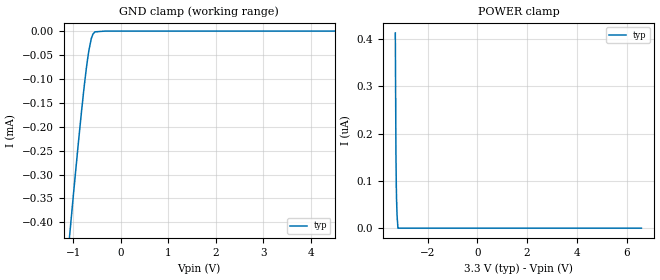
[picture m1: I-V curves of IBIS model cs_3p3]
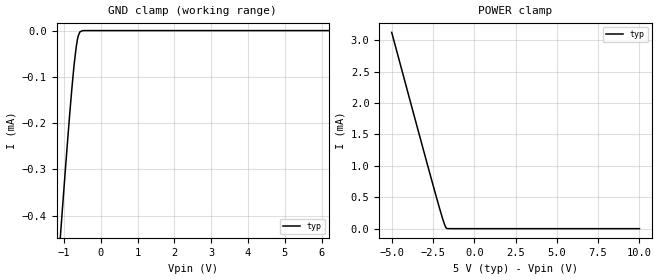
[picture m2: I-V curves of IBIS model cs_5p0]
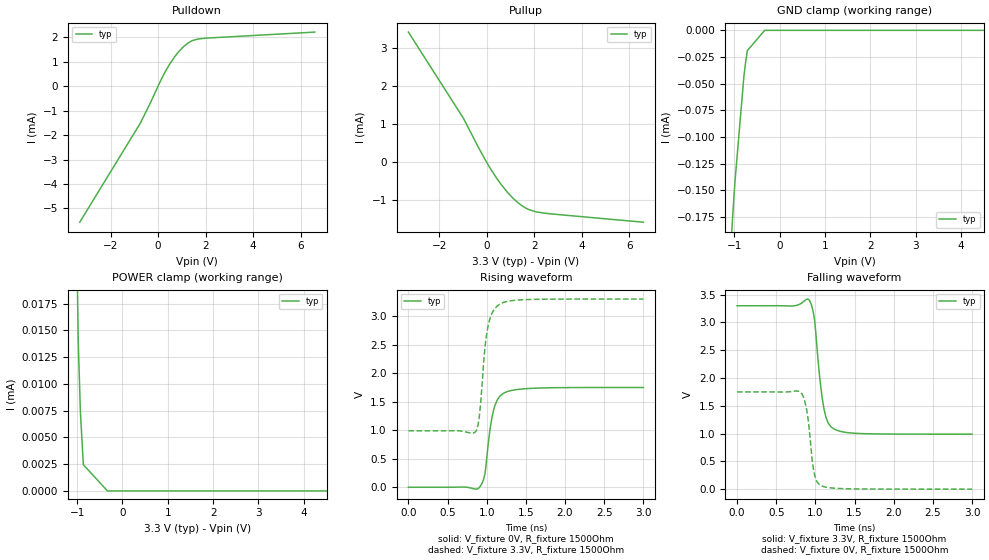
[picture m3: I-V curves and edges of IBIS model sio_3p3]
|Texas Instruments Incorporated
|LM70 SPI/MICROWIRE 10-Bit plus Sign Digital Temperature Sensor
|Marketing part#   Digital Voltage Range   Package-type   #pins
|LM70CIMM-3   2.65-5.5   VSSOP   8
|LM70CIMM-3/NOPB   2.65-5.5   VSSOP   8
|LM70CIMM-5   2.65-5.5   VSSOP   8
|LM70CIMM-5/NOPB   2.65-5.5   VSSOP   8
|LM70CIMMX-3   2.65-5.5   VSSOP   8
|LM70CIMMX-3/NOPB   2.65-5.5   VSSOP   8
|LM70CIMMX-5/NOPB   2.65-5.5   VSSOP   8
|LM70CILD-3/NOPB   2.65-5.5   WSON   8
|LM70CILD-5/NOPB   2.65-5.5   WSON   8
|LM70CILDX-3/NOPB   2.65-5.5   WSON   8
[IBIS Ver]   4.1
[File name]   lm70.ibs
[File Rev]   1.0
[Date]   10/25/2016
[Source]
| Texas Instruments Incorporated.
| Analog-eLab Design Center, HPA
| 12500 TI Blvd
| Dallas, TX -75243
[Notes]   Revision History:
| Rev 1.0: 10/25/2016
| - Initial version of the model
| - Model generated from simulations in SPECTRE
| - Model matched to SPICE simulation
| - C_comp although listed in numerical order of value are
|   obtained from varying PVT conditions. For PVT conditions for
|   each specific value refer the buffer description under
|   respective [Model]. IBIS model user is responsible for using
|   appropriate C_comp to simulate for Signal Integrity.
| - Only Typical corners are modeled.
[Disclaimer]
| This model is designed as an aid for customers of Texas Instruments.
| TI and its licensors and suppliers make no warranties, either expressed
| or implied, with respect to this  model, including the warranties of
| merchantability or fitness for a particular purpose. The model is
| provided solely on an "as is" basis. The entire risk as to its quality
| and performance is with the customer.
[Copyright]
(C) Copyright 2016 Texas Instruments Incorporated.All rights reserved.
|   LM70DGK
[Component]   LM70DGK
[Manufacturer]   TI
[Package]   |8 VSSOP - DGK Package
|   typ   min   max
R_pkg   0.5   na   na
L_pkg   1n   na   na
C_pkg   .5p   na   na
[Pin]  signal_name   model_name   R_pin   L_pin   C_pin
1   SI/O   sio   na   na   na
2   SC   cs   na   na   na
3   NC   nc   na   na   na
4   GND   gnd   na   na   na
5   V+   power   na   na   na
6   NC   nc   na   na   na
7   _CS   cs   na   na   na
8   NC   nc   na   na   na
|   LM70NGK
[Component]   LM70NGK
[Manufacturer]   TI
[Package]   |8 WSON - NGK Package
|   typ   min   max
R_pkg   0.5   na   na
L_pkg   1n   na   na
C_pkg   .5p   na   na
[Pin]  signal_name   model_name   R_pin   L_pin   C_pin
1   SI/O   sio   na   na   na
2   NC   nc   na   na   na
3   SC   cs   na   na   na
4   NC   nc   na   na   na
5   V+   power   na   na   na
6   NC   nc   na   na   na
7   GND   gnd   na   na   na
8   _CS   cs   na   na   na
|   Model Selectors
[Model Selector] cs
cs_3p3   3.3  digital input
cs_5p0   5.0  digital input
[Model Selector] sio
sio_3p3   3.3  digital 3-state
sio_5p0   5.0  digital 3-state
| Models and submodels in the file (4): cs_3p3 (Input), cs_5p0 (Input), sio_3p3 (3-state), sio_5p0 (3-state)
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|   cs_3p3 Model
[Model]   cs_3p3
Model_type   Input
Vinl = 0.99
Vinh = 2.31
|   typ   min   max
|   (nom PVT)   (fast PVT)   (slow PVT)
C_comp   3.012e-14   2.938e-14   3.092e-14
| Where nom  PVT is Nominal Process, 3.3V, 27C
|   Fast PVT is Strong Process,  3.6V, -55C
|   Slow PVT is Weak Process,   2.65V, 150C
[Model spec]
|subparameter
Vinl   0.99   0.795   1.08
Vinh   2.31   1.855   2.52
[Voltage Range]   3.3   2.65   3.6
|Junction Temperature
[Temperature Range]   27   150   -55
[Power Clamp Reference]   3.3   2.65   3.6
[GND Clamp Reference]   0   0   0
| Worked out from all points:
|   GND clamp passes 1 mA (typ) near -1.60 V on its own axis
[GND Clamp]
|   Voltage   I(typ)   I(min)   I(max)
-3.3V     -2.937mA   NA         NA
-1.133V   -487uA     NA         NA
-1.01V    -355.5uA   NA         NA
-907.5mV  -248.1uA   NA         NA
-821.7mV  -162.8uA   NA         NA
-754.8mV  -101.8uA   NA         NA
-693.6mV  -54.41uA   NA         NA
-669.9mV  -39.22uA   NA         NA
-620.4mV  -15.3uA    NA         NA
-587.4mV  -6.359uA   NA         NA
-544.5mV  -1.581uA   NA         NA
6.6V      0A         NA         NA
[POWER Clamp]
|   Voltage   I(typ)   I(min)   I(max)
-3.3V     412.6nA    NA         NA
-3.275V   157.6nA    NA         NA
-3.26V    90.42nA    NA         NA
-3.251V   61.75nA    NA         NA
-3.232V   29.85nA    NA         NA
-3.221V   19.65nA    NA         NA
-3.21V    12.98nA    NA         NA
-3.196V   0A         NA         NA
6.6V      0A         NA         NA
|   cs_5p0 Model
[Model]   cs_5p0
Model_type   Input
Vinl = 1.5
Vinh = 3.5
|   typ   min   max
|   (nom PVT)   (fast PVT)   (slow PVT)
C_comp   2.774e-14   2.762e-14   2.918e-14
| Where nom  PVT is Nominal Process, 5V, 27C
|   Fast PVT is Strong Process,  5.5V, -55C
|   Slow PVT is Weak Process,   4.5V, 150C
[Model spec]
|subparameter
Vinl   1.5   1.35   1.65
Vinh   3.5   3.15   3.85
[Voltage Range]   5   4.5   5.5
|Junction Temperature
[Temperature Range]   27   150   -55
[Power Clamp Reference]   5   4.5   5.5
[GND Clamp Reference]   0   0   0
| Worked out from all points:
|   GND clamp passes 1 mA (typ) near -1.60 V on its own axis
[GND Clamp]
|   Voltage   I(typ)   I(min)   I(max)
-5V       -4.886mA   NA         NA
-1.121V   -472.3uA   NA         NA
-1.046V   -391uA     NA         NA
-957.5mV  -298uA     NA         NA
-842mV    -180.8uA   NA         NA
-765mV    -109.1uA   NA         NA
-715.5mV  -68.88uA   NA         NA
-665mV    -35.38uA   NA         NA
-615mV    -12.89uA   NA         NA
-570mV    -3.513uA   NA         NA
-500mV    -306.2nA   NA         NA
10V       0A         NA         NA
[POWER Clamp]
|   Voltage   I(typ)   I(min)   I(max)
-5V       3.126mA    NA         NA
-3.322V   1.489mA    NA         NA
-2.275V   484.4uA    NA         NA
-1.893V   138.9uA    NA         NA
-1.745V   31.32uA    NA         NA
-1.675V   5.705uA    NA         NA
10V       0A         NA         NA
|   sio_3p3 Model
[Model]   sio_3p3
Model_type   3-state
Polarity   Non-Inverting
Vmeas = 1.65
Vref = 0
Cref = 80pF
Rref = 3300
|   typ   min   max
|   (nom PVT)   (fast PVT)   (slow PVT)
C_comp   3.680e-14   3.415e-14   4.057e-14
| Where nom  PVT is Nominal Process, 3.3V, 27C
|   Fast PVT is Strong Process,  3.6V, -55C
|   Slow PVT is Weak Process,   2.65V, 150C
[Voltage Range]   3.3   2.65   3.6
|Junction Temperature
[Temperature Range]   27   150   -55
[Pullup Reference]   3.3   2.65   3.6
[Pulldown Reference]   0   0   0
[Power Clamp Reference]   3.3   2.65   3.6
[GND Clamp Reference]   0   0   0
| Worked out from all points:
|   slope of the pulldown table from 0 to 0.495 V, typ, clamps not added: 545 ohm
|   slope of the pullup table from 0 to 0.495 V, typ, clamps not added: 1.02 kohm
|   GND clamp passes 1 mA (typ) near -1.30 V on its own axis
|   POWER clamp passes 1 mA (typ) near -1.29 V on its own axis
|   falling waveform, V_fixture 3.3V, R_fixture 1500Ohm: 20-80 % time 105ps typ, NA min, NA max; typ from 3.3 V to 0.99 V
|   rising waveform, V_fixture 0V, R_fixture 1500Ohm: 20-80 % time 110ps typ, NA min, NA max; typ from 0 V to 1.75 V
|   rising waveform, V_fixture 3.3V, R_fixture 1500Ohm: 20-80 % time 97.9ps typ, NA min, NA max; typ from 0.99 V to 3.3 V
|   falling waveform, V_fixture 0V, R_fixture 1500Ohm: 20-80 % time 85.2ps typ, NA min, NA max; typ from 1.75 V to 0 V
[Pulldown]
|   Voltage   I(typ)   I(min)   I(max)
-3.3V     -5.568mA   NA         NA
-734.8mV  -1.486mA   NA         NA
-330mV    -689.9uA   NA         NA
102.6mV   218.6uA    NA         NA
417.9mV   792.2uA    NA         NA
762.4mV   1.289mA    NA         NA
1.11V     1.655mA    NA         NA
1.439V    1.866mA    NA         NA
1.82V     1.952mA    NA         NA
6.6V      2.219mA    NA         NA
[GND Clamp]
|   Voltage   I(typ)   I(min)   I(max)
-3.3V     -52.66mA   NA         NA
-1.151V   -251.3uA   NA         NA
-1.005V   -153.7uA   NA         NA
-980.1mV  -138.9uA   NA         NA
-790.8mV  -43.91uA   NA         NA
-755.7mV  -31.22uA   NA         NA
-713.6mV  -19.04uA   NA         NA
-330mV    -2.582nA   NA         NA
6.6V      0A         NA         NA
[Pullup]
|   Voltage   I(typ)   I(min)   I(max)
-3.3V     3.415mA    NA         NA
-1.003V   1.174mA    NA         NA
-330mV    367.1uA    NA         NA
171.5mV   -182uA     NA         NA
495mV     -486.5uA   NA         NA
850.8mV   -771.3uA   NA         NA
1.301V    -1.053mA   NA         NA
1.65V     -1.204mA   NA         NA
2.155V    -1.309mA   NA         NA
6.6V      -1.573mA   NA         NA
[POWER Clamp]
|   Voltage   I(typ)   I(min)   I(max)
-3.3V     61.22mA    NA         NA
-1.136V   60.6uA     NA         NA
-974.4mV  13.92uA    NA         NA
-927.3mV  7.385uA    NA         NA
-862mV    2.447uA    NA         NA
-330mV    0A         NA         NA
6.6V      0A         NA         NA
[Ramp]
R_load = 1500
|   typ   min   max
dV/dt_r   1.04972/1.09729e-10   NA   NA
dV/dt_f   1.38621/1.05391e-10   NA   NA
[Falling Waveform]
V_fixture = 3.3V
V_fixture_min = 2.65V
V_fixture_max = 3.6V
R_fixture = 1500Ohm
|   Time   V(typ)   V(min)   V(max)
0s        3.3V       NA         NA
710.6ps   3.296V     NA         NA
923ps     3.402V     NA         NA
990.5ps   3.04V      NA         NA
1.048ns   2.123V     NA         NA
1.107ns   1.465V     NA         NA
1.165ns   1.189V     NA         NA
1.231ns   1.089V     NA         NA
1.559ns   1.002V     NA         NA
3ns       989.7mV    NA         NA
[Rising Waveform]
V_fixture = 0V
V_fixture_min = 0V
V_fixture_max = 0V
R_fixture = 1500Ohm
|   Time   V(typ)   V(min)   V(max)
0s        1.116nV    NA         NA
904.2ps   -7.198mV   NA         NA
945.4ps   85.74mV    NA         NA
977.1ps   233.6mV    NA         NA
1.033ns   919.7mV    NA         NA
1.088ns   1.354V     NA         NA
1.134ns   1.531V     NA         NA
1.231ns   1.66V      NA         NA
1.621ns   1.737V     NA         NA
3ns       1.75V      NA         NA
[Rising Waveform]
V_fixture = 3.3V
V_fixture_min = 2.65V
V_fixture_max = 3.6V
R_fixture = 1500Ohm
|   Time   V(typ)   V(min)   V(max)
0s        989.6mV    NA         NA
865.8ps   989.1mV    NA         NA
904.2ps   1.223V     NA         NA
923ps     1.478V     NA         NA
977.1ps   2.447V     NA         NA
1.005ns   2.738V     NA         NA
1.065ns   3.044V     NA         NA
1.165ns   3.209V     NA         NA
1.499ns   3.291V     NA         NA
3ns       3.3V       NA         NA
[Falling Waveform]
V_fixture = 0V
V_fixture_min = 0V
V_fixture_max = 0V
R_fixture = 1500Ohm
|   Time   V(typ)   V(min)   V(max)
0s        1.75V      NA         NA
810.4ps   1.747V     NA         NA
849.3ps   1.655V     NA         NA
886.3ps   1.45V      NA         NA
923ps     1.072V     NA         NA
960.7ps   506.6mV    NA         NA
990.5ps   260mV      NA         NA
1.033ns   110mV      NA         NA
1.088ns   54.73mV    NA         NA
3ns       29.9uV     NA         NA
